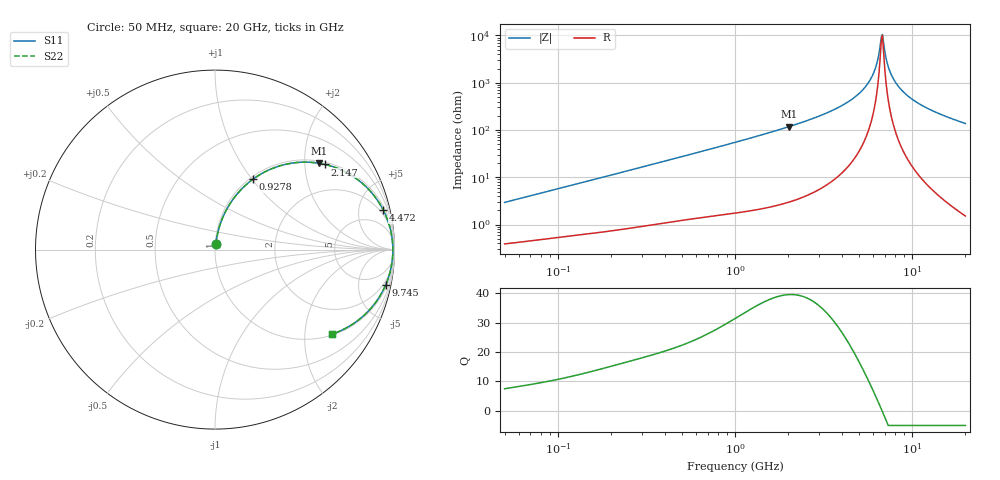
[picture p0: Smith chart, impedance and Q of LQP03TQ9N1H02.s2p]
!Murata Part Number: LQP03TQ9N1H02
!These Parameters are Measured in Series Mode Connection
!  o--[Z]--o
!Port1  Port2
!  o-------o
!Freq. Start=50[MHz] Stop=20[GHz], 401[Steps]
# Hz S RI R 50
!Freq.(Hz) S11(Real) S11(Imag) S21(Real) S21(Imag) S12(Real) S12(Imag) S22(Real) S22(Imag)
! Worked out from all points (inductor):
!   401 points, 50 MHz to 20 GHz, reference 50 ohm
!   read as one part in series: L = 9.19 nH near 51.52 MHz
!   highest Q = 39.5 at 2.022 GHz (marker M1), where L = 9.3 nH
!   self-resonance near 6.701 GHz
!   S11 on the Smith chart (normalised r, x): 50 MHz: 1.01, +0.06; 927.8 MHz: 1.03, +1.01; 2.147 GHz: 1.06, +2.54; 4.472 GHz: 1.38, +8.42; 9.745 GHz: 1.39, -9.63; 20 GHz: 1.03, -2.75
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5e7  0.00471 0.0289  0.9953 -0.0289  0.9953 -0.0289  0.00471 0.0289
1.364002e8  0.0118 0.0753  0.9882 -0.0753  0.9882 -0.0753  0.0118 0.0753
3.721004e8  0.049 0.1919  0.951 -0.1919  0.951 -0.1919  0.049 0.1919
9.278425e8  0.212 0.3925  0.788 -0.3925  0.788 -0.3925  0.212 0.3925
1e9  0.2375 0.4099  0.7625 -0.4099  0.7625 -0.4099  0.2375 0.4099
2.021818e9  0.5806 0.481  0.4194 -0.481  0.4194 -0.481  0.5806 0.481
2.146657e9  0.6145 0.4742  0.3855 -0.4742  0.3855 -0.4742  0.6145 0.4742
2.728004e9  0.7443 0.4231  0.2557 -0.4231  0.2557 -0.4231  0.7443 0.4231
3.572216e9  0.8659 0.325  0.1341 -0.325  0.1341 -0.325  0.8659 0.325
4.472136e9  0.9378 0.22  0.0622 -0.22  0.0622 -0.22  0.9378 0.22
5.273168e9  0.9714 0.1349  0.0286 -0.1349  0.0286 -0.1349  0.9714 0.1349
5.856089e9  0.9842 0.0788  0.0158 -0.0788  0.0158 -0.0788  0.9842 0.0788
6.217679e9  0.9886 0.0463  0.0114 -0.0463  0.0114 -0.0463  0.9886 0.0463
6.601595e9  0.9907 0.0136  0.00929 -0.0136  0.00929 -0.0136  0.9907 0.0136
6.701223e9  0.9909 0.00545  0.00909 -0.00545  0.00909 -0.00545  0.9909 0.00545
6.905011e9  0.9909 -0.0109  0.00911 0.0109  0.00911 0.0109  0.9909 -0.0109
7.222371e9  0.9898 -0.0354  0.0102 0.0354  0.0102 0.0354  0.9898 -0.0354
7.442007e9  0.9885 -0.0518  0.0115 0.0518  0.0115 0.0518  0.9885 -0.0518
8.264682e9  0.9793 -0.1086  0.0207 0.1086  0.0207 0.1086  0.9793 -0.1086
9.745021e9  0.9514 -0.1955  0.0486 0.1955  0.0486 0.1955  0.9514 -0.1955
1.314879e10  0.8586 -0.3382  0.1414 0.3382  0.1414 0.3382  0.8586 -0.3382
2e10  0.6522 -0.4708  0.3478 0.4708  0.3478 0.4708  0.6522 -0.4708
